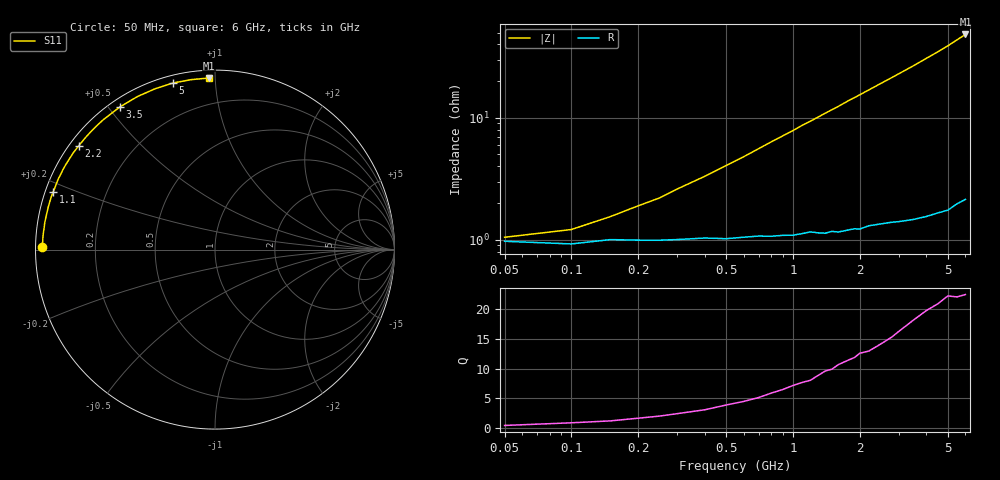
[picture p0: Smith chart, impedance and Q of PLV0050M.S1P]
! Infineon Technologies  Discrete & RF Semiconductors
! BAR 64-04W /-05W /-06W
! Si PIN Diode in SOT323
! IF = 50 mA
! S-Parameters:  October  2008
# GHz  S  MA  R  50
!  f  S11
! GHz  MAG  ANG
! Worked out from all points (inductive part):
!   34 points, 50 MHz to 6 GHz, reference 50 ohm
!   read as one part to ground: L = 1.25 nH near 400 MHz
!   highest Q = 22.5 at 6 GHz (marker M1), where L = 1.28 nH
!   S11 on the Smith chart (normalised r, x): 50 MHz: 0.02, +0.01; 1.1 GHz: 0.02, +0.17; 2.2 GHz: 0.03, +0.34; 3.5 GHz: 0.03, +0.53; 5 GHz: 0.03, +0.78; 6 GHz: 0.04, +0.96
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0.05  0.9619 179.1
0.1  0.9637 178.2
0.15  0.9607 177.3
0.2  0.9611 176.3
0.25  0.9612 175.5
0.3  0.9608 174.5
0.4  0.9597 172.8
0.5  0.9603 171.0
0.6  0.9593 169.3
0.8  0.9588 165.7
1  0.9583 162.3
1.1  0.9574 160.5
1.2  0.9562 158.9
1.4  0.9577 155.5
1.6  0.9573 152.3
1.8  0.9561 148.9
1.9  0.9557 147.4
2  0.9563 145.8
2.2  0.9543 142.7
2.4  0.9541 139.6
2.6  0.954 136.6
3  0.9545 130.8
3.5  0.9554 123.8
4  0.9559 116.9
4.5  0.9562 110.5
5  0.9574 104.2
5.5  0.9562 97.9
6  0.9566 92.1
